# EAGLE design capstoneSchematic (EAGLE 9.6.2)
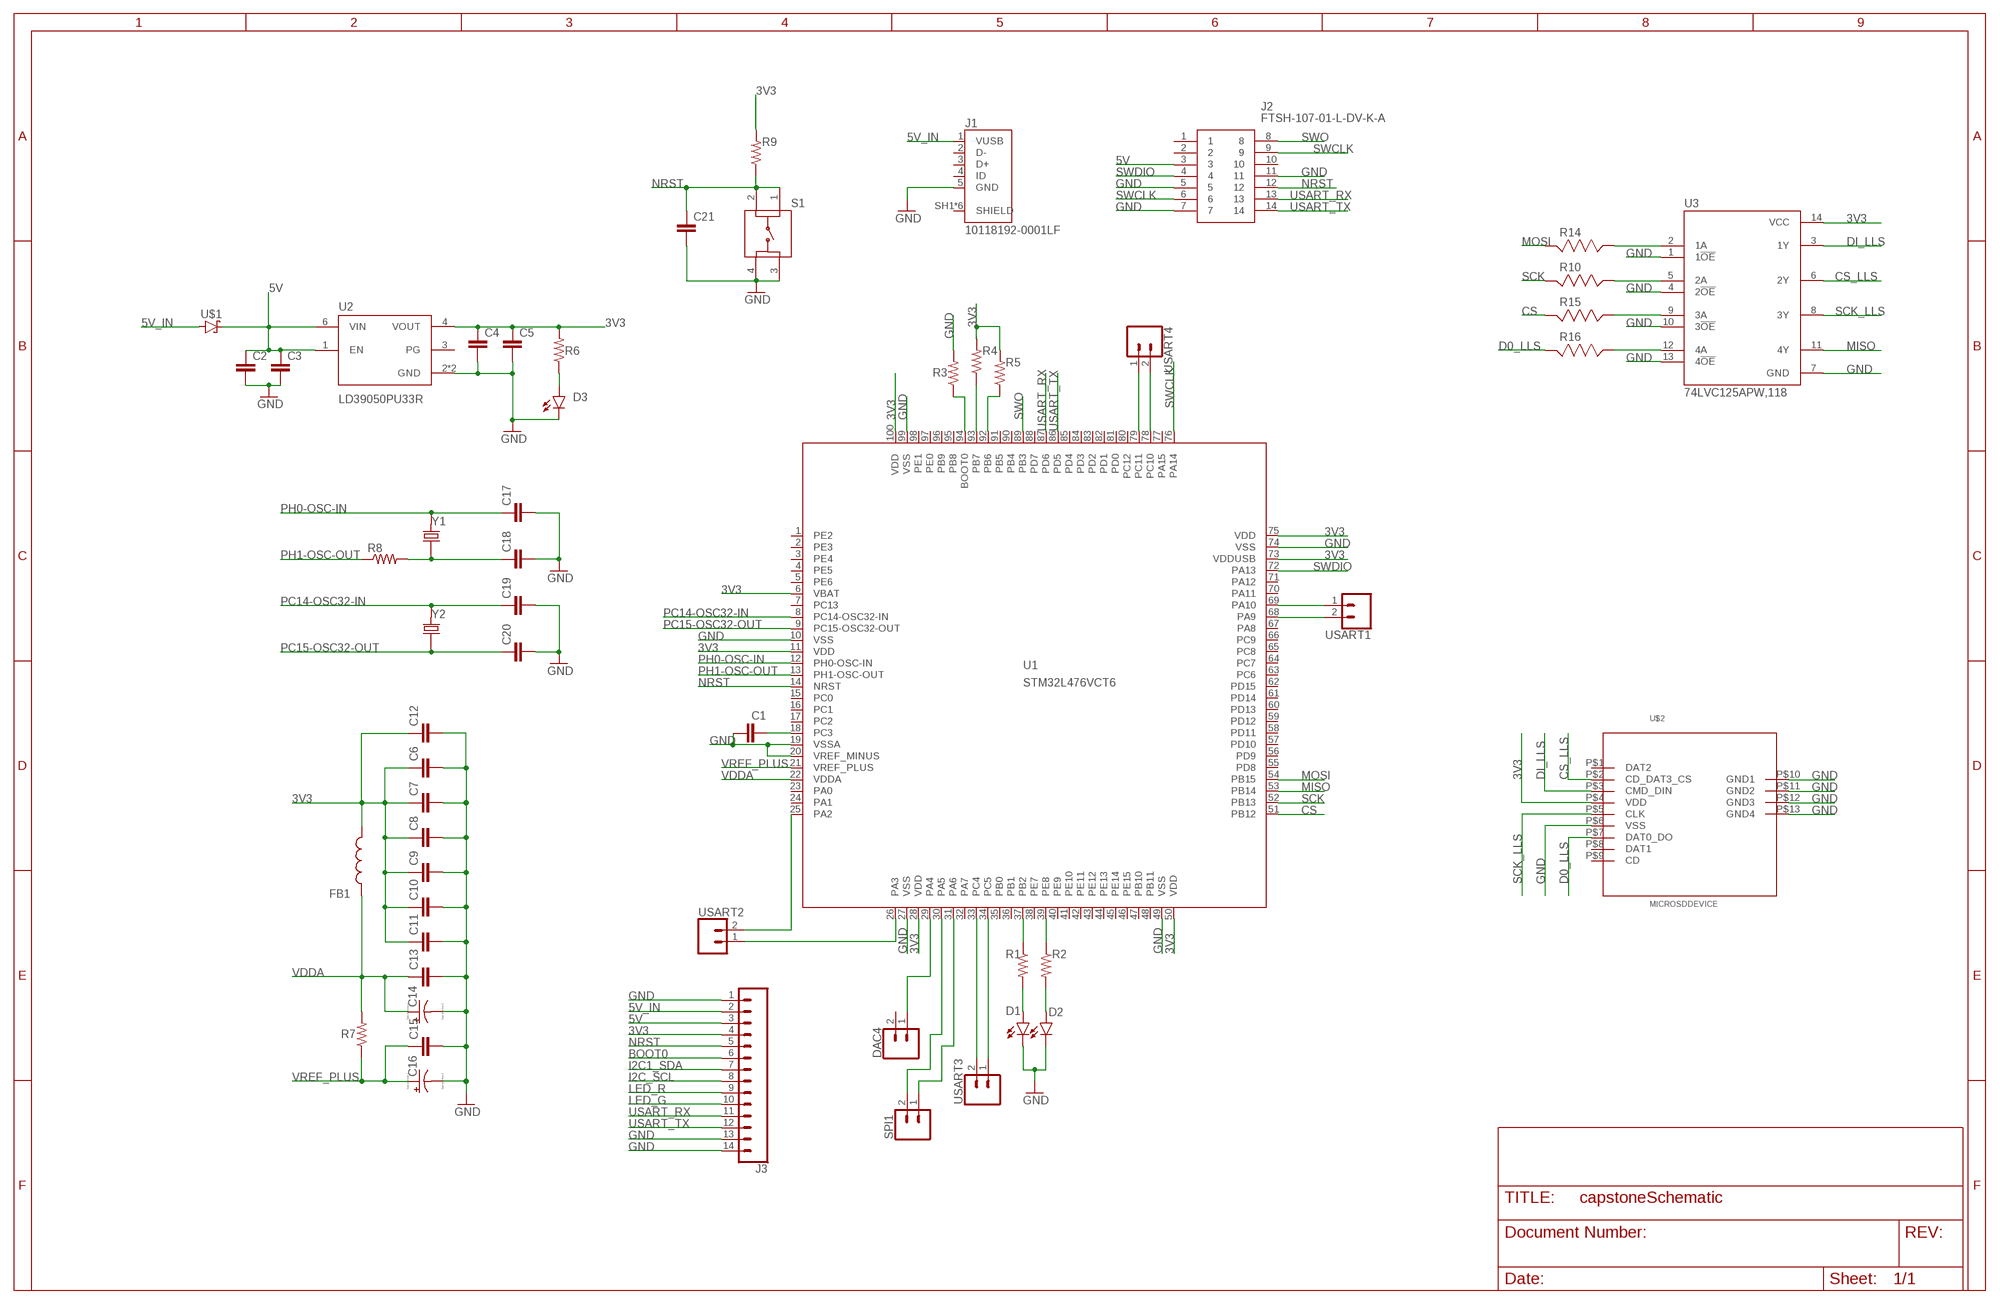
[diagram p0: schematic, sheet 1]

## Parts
C1  CC0603KRX5R7BB105  [CAPC1608X90]
C2  CC0603KRX5R7BB105  [CAPC1608X90]
C3  CC0402KRX7R7BB104  [CAPC1005X55N]
C4  CC0603KRX5R7BB105  [CAPC1608X90]
C5  CC0402KRX7R7BB104  [CAPC1005X55N]
C6  CC0402KRX7R7BB104  [CAPC1005X55N]
C7  CC0402KRX7R7BB104  [CAPC1005X55N]
C8  CC0402KRX7R7BB104  [CAPC1005X55N]
C9  CC0402KRX7R7BB104  [CAPC1005X55N]
C10  CC0402KRX7R7BB104  [CAPC1005X55N]
C11  CC0402KRX7R7BB104  [CAPC1005X55N]
C12  CC0603KRX5R7BB105  [CAPC1608X90]
C13  CC0402KRX7R7BB104  [CAPC1005X55N]
C14  TAJA105K016RNJ  [CAPPM3216X180N]
C15  CC0402KRX7R7BB104  [CAPC1005X55N]
C16  TAJA105K016RNJ  [CAPPM3216X180N]
C17  CC0402JRNPO9BN200  [CAPC1005X55N]
C18  CC0402JRNPO9BN200  [CAPC1005X55N]
C19  CC0402CRNPO9BN4R7  [CAPC1005X55N]
C20  CC0402CRNPO9BN4R7  [CAPC1005X55N]
C21  CC0402KRX7R7BB104  [CAPC1005X55N]
D1  SML-P12MTT86  [LED_SML-P11UTT86R]
D2  SML-P12MTT86  [LED_SML-P11UTT86R]
D3  SML-P12MTT86  [LED_SML-P11UTT86R]
DAC4  CONN_02  [1X02]
FB1  BK1608HS601-T  [BEADC1608X95N]
J1  10118192-0001LF  [AMPHENOL_10118192-0001LF]
J2  FTSH-107-01-L-DV-K-A  [FTSH10701LDVKA]
J3  CONN_14  [1X14]
R1  RC0402FR-071KL  [RESC1005X40N]
R2  RC0402FR-071KL  [RESC1005X40N]
R3  RC0402FR-071KL  [RESC1005X40N]
R4  RC0402FR-071KL  [RESC1005X40N]
R5  RC0402FR-071KL  [RESC1005X40N]
R6  RC0402FR-071KL  [RESC1005X40N]
R7  RC0402FR-071KL  [RESC1005X40N]
R8  RC0402FR-072KL  [RESC1005X40N]
R9  RC0402FR-0710KL  [RESC1005X40N]
R10  RC0402FR-073K3L  [RESC1005X40]
R14  RC0402FR-073K3L  [RESC1005X40]
R15  RC0402FR-073K3L  [RESC1005X40]
R16  RC0402FR-073K3L  [RESC1005X40]
S1  LL3301FF065QJ  [LL3301FF065QJ]
SPI1  CONN_02  [1X02]
U1  STM32L476VCT6  [LQFP100_14X14]
U2  LD39050PU33R  [SON95P300X300X100-7N]
U3  74LVC125APW,118  [IC_74LVC125APW,118]
U$1  STPS1L30A  [DIOM5226X223N]
U$2  MICROSDDEVICE  [MICROSD]
USART1  CONN_02  [1X02]
USART2  CONN_02  [1X02]
USART3  CONN_02  [1X02]
USART4  CONN_02  [1X02]
Y1  ABLS-8.000MHZ-B2-T  [XTAL_ABLS-8.000MHZ-B2-T]
Y2  ECS-.327-12.5-12QS-TR  [XTAL_ECS-.327-12.5-12QS-TR]

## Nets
3V3: C4.1 C5.1 C6.1 C7.1 C8.1 C9.1 C10.1 C11.1 C12.1 FB1.2 J3.4 R4.2 R5.2 R6.2 R9.2 U1.6(VBAT) U1.11(VDD) U1.28(VDD) U1.50(VDD) U1.73(VDDUSB) U1.75(VDD) U1.100(VDD) U2.4(VOUT) U3.14(VCC) U$2.P$4(VDD)
5V: C2.1 C3.1 J2.3 J3.3 U2.1(EN) U2.6(VIN) U$1.1(C)
5V_IN: J1.1(VUSB) J3.2 U$1.2(A)
BOOT0: J3.6
CS: R15.1 U1.51(PB12)
CS_LLS: U3.6(2Y) U$2.P$2(CD_DAT3_CS)
D0_LLS: R16.1 U$2.P$7(DAT0_DO)
DI_LLS: U3.3(1Y) U$2.P$3(CMD_DIN)
GND: C1.1 C2.2 C3.2 C4.2 C5.2 C6.2 C7.2 C8.2 C9.2 C10.2 C11.2 C12.2 C13.2 C14.C(-) C15.2 C16.C(-) C17.2 C18.2 C19.2 C20.2 C21.2 D1.C D2.C D3.C J1.5(GND) J2.5 J2.7 J2.11 J3.1 J3.13 J3.14 R3.2 S1.3 S1.4 U1.10(VSS) U1.19(VSSA) U1.20(VREF_MINUS) U1.27(VSS) U1.49(VSS) U1.74(VSS) U1.99(VSS) U2.2(GND) U2.7(GND) U3.1(1!OE) U3.4(2!OE) U3.7(GND) U3.10(3!OE) U3.13(4!OE) U$2.P$6(VSS) U$2.P$10(GND1) U$2.P$11(GND2) U$2.P$12(GND3) U$2.P$13(GND4)
I2C1_SDA: J3.7
I2C_SCL: J3.8
LED_G: J3.10
LED_R: J3.9
MISO: U1.53(PB14) U3.11(4Y)
MOSI: R14.1 U1.54(PB15)
N$1: R2.1 U1.39(PE8)
N$2: R1.1 U1.37(PB2)
N$3: D1.A R1.2
N$4: D2.A R2.2
N$5: R3.1 U1.94(BOOT0)
N$6: R4.1 U1.93(PB7)
N$7: R5.1 U1.92(PB6)
N$8: D3.A R6.1
N$9: U1.33(PC4) USART3.2
N$10: C1.2 U1.18(PC3)
N$11: U1.34(PC5) USART3.1
N$12: C18.1 R8.2 Y1.1
N$13: R14.2 U3.2(1A)
N$14: U1.78(PC10) USART4.2
N$15: DAC4.1 U1.29(PA4)
N$16: U1.79(PC11) USART4.1
N$17: SPI1.2 U1.30(PA5)
N$18: SPI1.1 U1.31(PA6)
N$19: U1.69(PA10) USART1.1
N$20: U1.68(PA9) USART1.2
N$22: U1.25(PA2) USART2.2
N$23: U1.26(PA3) USART2.1
N$24: R10.2 U3.5(2A)
N$25: R15.2 U3.9(3A)
N$26: R16.2 U3.12(4A)
NRST: C21.1 J2.12 J3.5 R9.1 S1.1 S1.2 U1.14(NRST)
PC14-OSC32-IN: C19.1 U1.8(PC14-OSC32-IN) Y2.2
PC15-OSC32-OUT: C20.1 U1.9(PC15-OSC32-OUT) Y2.1
PH0-OSC-IN: C17.1 U1.12(PH0-OSC-IN) Y1.2
PH1-OSC-OUT: R8.1 U1.13(PH1-OSC-OUT)
SCK: R10.1 U1.52(PB13)
SCK_LLS: U3.8(3Y) U$2.P$5(CLK)
SWCLK: J2.6 J2.9 U1.76(PA14)
SWDIO: J2.4 U1.72(PA13)
SWO: J2.8 U1.89(PB3)
USART_RX: J2.13 J3.11 U1.87(PD6)
USART_TX: J2.14 J3.12 U1.86(PD5)
VDDA: C13.1 C14.A(+) FB1.1 R7.2 U1.22(VDDA)
VREF_PLUS: C15.1 C16.A(+) R7.1 U1.21(VREF_PLUS)
Unconnected: DAC4.2 J1.2(D-) J1.3(D+) J1.4(ID) J1.SH1(SHIELD) J1.SH2(SHIELD) J1.SH3(SHIELD) J1.SH4(SHIELD) J1.SH5(SHIELD) J1.SH6(SHIELD) J2.1 J2.2 J2.10 U1.1(PE2) U1.2(PE3) U1.3(PE4) U1.4(PE5) U1.5(PE6) U1.7(PC13) U1.15(PC0) U1.16(PC1) U1.17(PC2) U1.23(PA0) U1.24(PA1) U1.32(PA7) U1.35(PB0) U1.36(PB1) U1.38(PE7) U1.40(PE9) U1.41(PE10) U1.42(PE11) U1.43(PE12) U1.44(PE13) U1.45(PE14) U1.46(PE15) U1.47(PB10) U1.48(PB11) U1.55(PD8) U1.56(PD9) U1.57(PD10) U1.58(PD11) U1.59(PD12) U1.60(PD13) U1.61(PD14) U1.62(PD15) U1.63(PC6) U1.64(PC7) U1.65(PC8) U1.66(PC9) U1.67(PA8) U1.70(PA11) U1.71(PA12) U1.77(PA15) U1.80(PC12) U1.81(PD0) U1.82(PD1) U1.83(PD2) U1.84(PD3) U1.85(PD4) U1.88(PD7) U1.90(PB4) U1.91(PB5) U1.95(PB8) U1.96(PB9) U1.97(PE0) U1.98(PE1) U2.3(PG) U$2.P$1(DAT2) U$2.P$8(DAT1) U$2.P$9(CD)

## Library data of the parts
C1 C2 C4 C12 = ce-capstone:CC0603KRX5R7BB105: CAPACITOR CERAMIC, 1µF, 10V, X5R, 0603; Dielectric Characteristic:X5R; Capacitance:1µF; Capacitance Tolerance:± 10%; Voltage Rating:16V; Temperature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; DESCRIPTION: 1µF ±10% 16V Ceramic Capacitor X5R 0603 _1608 Metric_; DIGI-KEY_PART_NUMBER: 311-1444-1-ND; DIGI-KEY_PURCHASE_URL: https://www.digikey.com/product-detail/en/yageo/CC0603KRX5R7BB105/311-1444-1-ND/2833750?utm_source=snapeda&utm_medium=aggregator&utm_campaign=symbol; MF: Yageo; MP: CC0603KRX5R7BB105; PACKAGE: 0603 Yageo
C3 C5-C11 C13 C15 C21 = ce-capstone:CC0402KRX7R7BB104: .1UF 16V 10% 0402; DESCRIPTION: 0.1µF ±10% 16V Ceramic Capacitor X7R 0402 _1005 Metric_; DIGI-KEY_PART_NUMBER: 311-1338-1-ND; DIGI-KEY_PURCHASE_URL: https://www.digikey.com/product-detail/en/yageo/CC0402KRX7R7BB104/311-1338-1-ND/2103122?utm_source=snapeda&utm_medium=aggregator&utm_campaign=symbol; MF: Yageo; MP: CC0402KRX7R7BB104; PACKAGE: 0402 Yageo
C14 C16 = ce-capstone:TAJA105K016RNJ: Capacitor tantalum TAJ 1206 1uF 16V AVX 1uF SMD Solid MnO2 Tantalum Electrolytic Capacitor, 16 V dc +/-10%, TAJ Series; ALLIED_NUMBER: 70474975; ALLIED_PRICE-STOCK: https://www.alliedelec.com/avx-taja105k016r/70474975/; DESCRIPTION: Capacitor tantalum TAJ 1206 1uF 16V AVX 1uF SMD Solid MnO2 Tantalum Electrolytic Capacitor, 16 V dc +/-10%, TAJ Series; HEIGHT: 1.8mm; MANUFACTURER_NAME: AVX; MANUFACTURER_PART_NUMBER: TAJA105K016RNJ; MOUSER_PART_NUMBER: 581-TAJA105K016RNJ; MOUSER_PRICE-STOCK: https://www.mouser.com/Search/Refine.aspx?Keyword=581-TAJA105K016R; RS_PART_NUMBER: 6992804P; RS_PRICE-STOCK: http://uk.rs-online.com/web/p/products/6992804P
C17 C18 = ce-capstone:CC0402JRNPO9BN200: CAPACITOR CERAMIC 20PF 50V, C0G, 0402; Dielectric Characteristic:C0G / NP0; Capacitance:20pF; Capacitance Tolerance:± 5%; Voltage Rating:50V; Capacitor Case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; DESCRIPTION: 20pF ±5% 50V Ceramic Capacitor C0G, NP0 0402 _1005 Metric_; DIGI-KEY_PART_NUMBER: 311-1417-1-ND; DIGI-KEY_PURCHASE_URL: https://www.digikey.com/product-detail/en/yageo/CC0402JRNPO9BN200/311-1417-1-ND/2833723?utm_source=snapeda&utm_medium=aggregator&utm_campaign=symbol; MF: Yageo; MP: CC0402JRNPO9BN200; PACKAGE: 0402 Yageo
C19 C20 = ce-capstone:CC0402CRNPO9BN4R7: 0402 4.7 pF 50 V ±0.25 pF Tolerance NP0 SMT Multilayer Ceramic Capacitor; DESCRIPTION: 4.7pF ±0.25pF 50V Ceramic Capacitor C0G, NP0 0402 _1005 Metric_; DIGI-KEY_PART_NUMBER: 311-1367-1-ND; DIGI-KEY_PURCHASE_URL: https://www.digikey.com/product-detail/en/yageo/CC0402CRNPO9BN4R7/311-1367-1-ND/2103151?utm_source=snapeda&utm_medium=aggregator&utm_campaign=symbol; MF: Yageo; MP: CC0402CRNPO9BN4R7; PACKAGE: 0402 Yageo
D1-D3 = ce-capstone:SML-P12MTT86: SML-P1 Series Red 0402 Clear 60 mcd 2 V Surface Mount PICOLED LED; AVAILABILITY: Unavailable; DESCRIPTION: Green 572nm LED Indication - Discrete 2V 0402 _1006 Metric_; MF: Rohm; MP: SML-P12MTT86; PACKAGE: 0402 Rohm; PRICE: None
DAC4 SPI1 USART1-USART4 = SparkFun-Connectors:CONN_02: Multi connection point. Often used as Generic Header-pin footprint for 0.1 inch spaced/style header connections
FB1 = ce-capstone:BK1608HS601-T: Ferrite Chip Bead(Lead Free); DESCRIPTION: Ferrite Chip Bead(Lead Free); HEIGHT: 0.95mm; MANUFACTURER_NAME: Taiyo Yuden; MANUFACTURER_PART_NUMBER: BK1608HS601-T
J1 = ce-capstone:10118192-0001LF: Single Port 5 Contact Horizontal Right Angle Shielded Micro B USB 2.0 Connector; AVAILABILITY: Unavailable; DESCRIPTION: USB - micro B USB 2.0 Receptacle Connector 5 Position Surface Mount, Right Angle; MF: Amphenol ICC; MP: 10118192-0001LF; PACKAGE: None; PRICE: None
J2 = ce-capstone:FTSH-107-01-L-DV-K-A: Headers & Wire Housings .050" Micro Terminal Strip Source: Datasheet; DESCRIPTION: Headers & Wire Housings .050" Micro Terminal Strip; HEIGHT: 5.97mm; MANUFACTURER_NAME: SAMTEC; MANUFACTURER_PART_NUMBER: FTSH-107-01-L-DV-K-A; MOUSER_PART_NUMBER: 200-FTSH10701LDVKA; MOUSER_PRICE-STOCK: https://www.mouser.com/Search/Refine.aspx?Keyword=200-FTSH10701LDVKA
J3 = SparkFun-Connectors:CONN_14: Multi connection point. Often used as Generic Header-pin footprint for 0.1 inch spaced/style header connections On any of the 0.1 inch spaced packages, you can populate with these: Break Away Headers - Straight (PRT-00116) Break Away Male Headers - Right Angle (PRT-00553) Female Headers (PRT-00115)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
R1-R7 = ce-capstone:RC0402FR-071KL: RES SMD 1k OHM 1% 1/16W 0402; DESCRIPTION: 510 Ohms ±1% 0.063W, 1/16W Chip Resistor 0402 _1005 Metric_ Moisture Resistant Thick Film; DIGI-KEY_PART_NUMBER: 311-510LRCT-ND; DIGI-KEY_PURCHASE_URL: https://www.digikey.com/product-detail/en/yageo/RC0402FR-07510RL/311-510LRCT-ND/729579?utm_source=snapeda&utm_medium=aggregator&utm_campaign=symbol; MF: Yageo; MP: RC0402FR-07510RL; PACKAGE: 1005 Panasonic Electronic Components
R8 = ce-capstone:RC0402FR-072KL: RES SMD 2k OHM 1% 1/16W 0402; DESCRIPTION: 510 Ohms ±1% 0.063W, 1/16W Chip Resistor 0402 _1005 Metric_ Moisture Resistant Thick Film; DIGI-KEY_PART_NUMBER: 311-510LRCT-ND; DIGI-KEY_PURCHASE_URL: https://www.digikey.com/product-detail/en/yageo/RC0402FR-07510RL/311-510LRCT-ND/729579?utm_source=snapeda&utm_medium=aggregator&utm_campaign=symbol; MF: Yageo; MP: RC0402FR-07510RL; PACKAGE: 1005 Panasonic Electronic Components
R9 = ce-capstone:RC0402FR-0710KL: RES SMD 10k OHM 1% 1/16W 0402; DESCRIPTION: 510 Ohms ±1% 0.063W, 1/16W Chip Resistor 0402 _1005 Metric_ Moisture Resistant Thick Film; DIGI-KEY_PART_NUMBER: 311-510LRCT-ND; DIGI-KEY_PURCHASE_URL: https://www.digikey.com/product-detail/en/yageo/RC0402FR-07510RL/311-510LRCT-ND/729579?utm_source=snapeda&utm_medium=aggregator&utm_campaign=symbol; MF: Yageo; MP: RC0402FR-07510RL; PACKAGE: 1005 Panasonic Electronic Components
R10 R14-R16 = RC0402FR-073K3L:RC0402FR-073K3L: RC Series 0402 0.063 W 3.3 kOhms ±1% ±100 ppm/°C SMT Thick Film Chip Resistor; MANUFACTURER: YAGEO
S1 = ce-capstone:LL3301FF065QJ: Pushbutton Switches 50mA 12VDC F065 7.0mm J-Lead Source: Datasheet; DESCRIPTION: Pushbutton Switches 50mA 12VDC F065 7.0mm J-Lead; HEIGHT: 7.3mm; MANUFACTURER_NAME: E-Switch; MANUFACTURER_PART_NUMBER: LL3301FF065QJ; MOUSER_PART_NUMBER: 612-LL3301FF065QJ; MOUSER_PRICE-STOCK: https://www.mouser.com/Search/Refine.aspx?Keyword=612-LL3301FF065QJ
U1 = ce-capstone:STM32L476V*: STM32L476VX LQFP100 Datasheet STM32L476XX; FARNELL: 2518171; FLASH: 256kB; SRAM: 128kB
U2 = ce-capstone:LD39050PU33R: LD39050 Series 500 mA 3.3 V Fixed Low Noise LDO Voltage Regulator - DFN-6; AVAILABILITY: Unavailable; DESCRIPTION: Linear Voltage Regulator IC 1 Output 500mA 6-DFN _3x3_; MF: STMicroelectronics; MP: LD39050PU33R; PACKAGE: DFN-6 STMicroelectronics; PRICE: None
U3 = 74LVC125APW_118:74LVC125APW,118: Check availability Check availability Check availability; AVAILABILITY: In Stock; CHECK_PRICES: https://www.snapeda.com/parts/74LVC125APW,118/Nexperia/view-part/?ref=eda; DESCRIPTION: Buffer, Non-Inverting 4 Element 1 Bit per Element 3-State Output 14-TSSOP; MF: Nexperia USA Inc.; MP: 74LVC125APW,118; PACKAGE: TSSOP14-14 Nexperia USA Inc.; PRICE: None; PURCHASE-URL: https://www.snapeda.com/api/url_track_click_mouser/?unipart_id=5248541&manufacturer=Nexperia USA Inc.&part_name=74LVC125APW,118&search_term=None; SNAPEDA_LINK: https://www.snapeda.com/parts/74LVC125APW,118/Nexperia/view-part/?ref=snap
U$1 = ce-capstone:STPS1L30A
U$2 = MicroSDFootprint:MICROSDDEVICE
Y1 = ce-capstone:ABLS-8.000MHZ-B2-T: Crystal 8MHz Â±20ppm (Tol) Â±50ppm (Stability) 18pF FUND 80Ohm 2-Pin HC-49/US SMD T/R; AVAILABILITY: Unavailable; DESCRIPTION: 8MHz ±20ppm Crystal 18pF 80 Ohms HC-49/US; MF: Abracon LLC; MP: ABLS-8.000MHZ-B2; PACKAGE: HC-49/US Abracon LLC; PRICE: None
Y2 = ce-capstone:ECS-.327-12.5-12QS-TR: SMD CRYSTAL 32.768 KHz; AVAILABILITY: Unavailable; DESCRIPTION: 32.768kHz ±20ppm Crystal 12.5pF 90 kOhms 2-SMD, No Lead; MF: ECS Inc.; MP: ECS-.327-12.5-12QS-TR; PACKAGE: SMD-2 ECS International; PRICE: None

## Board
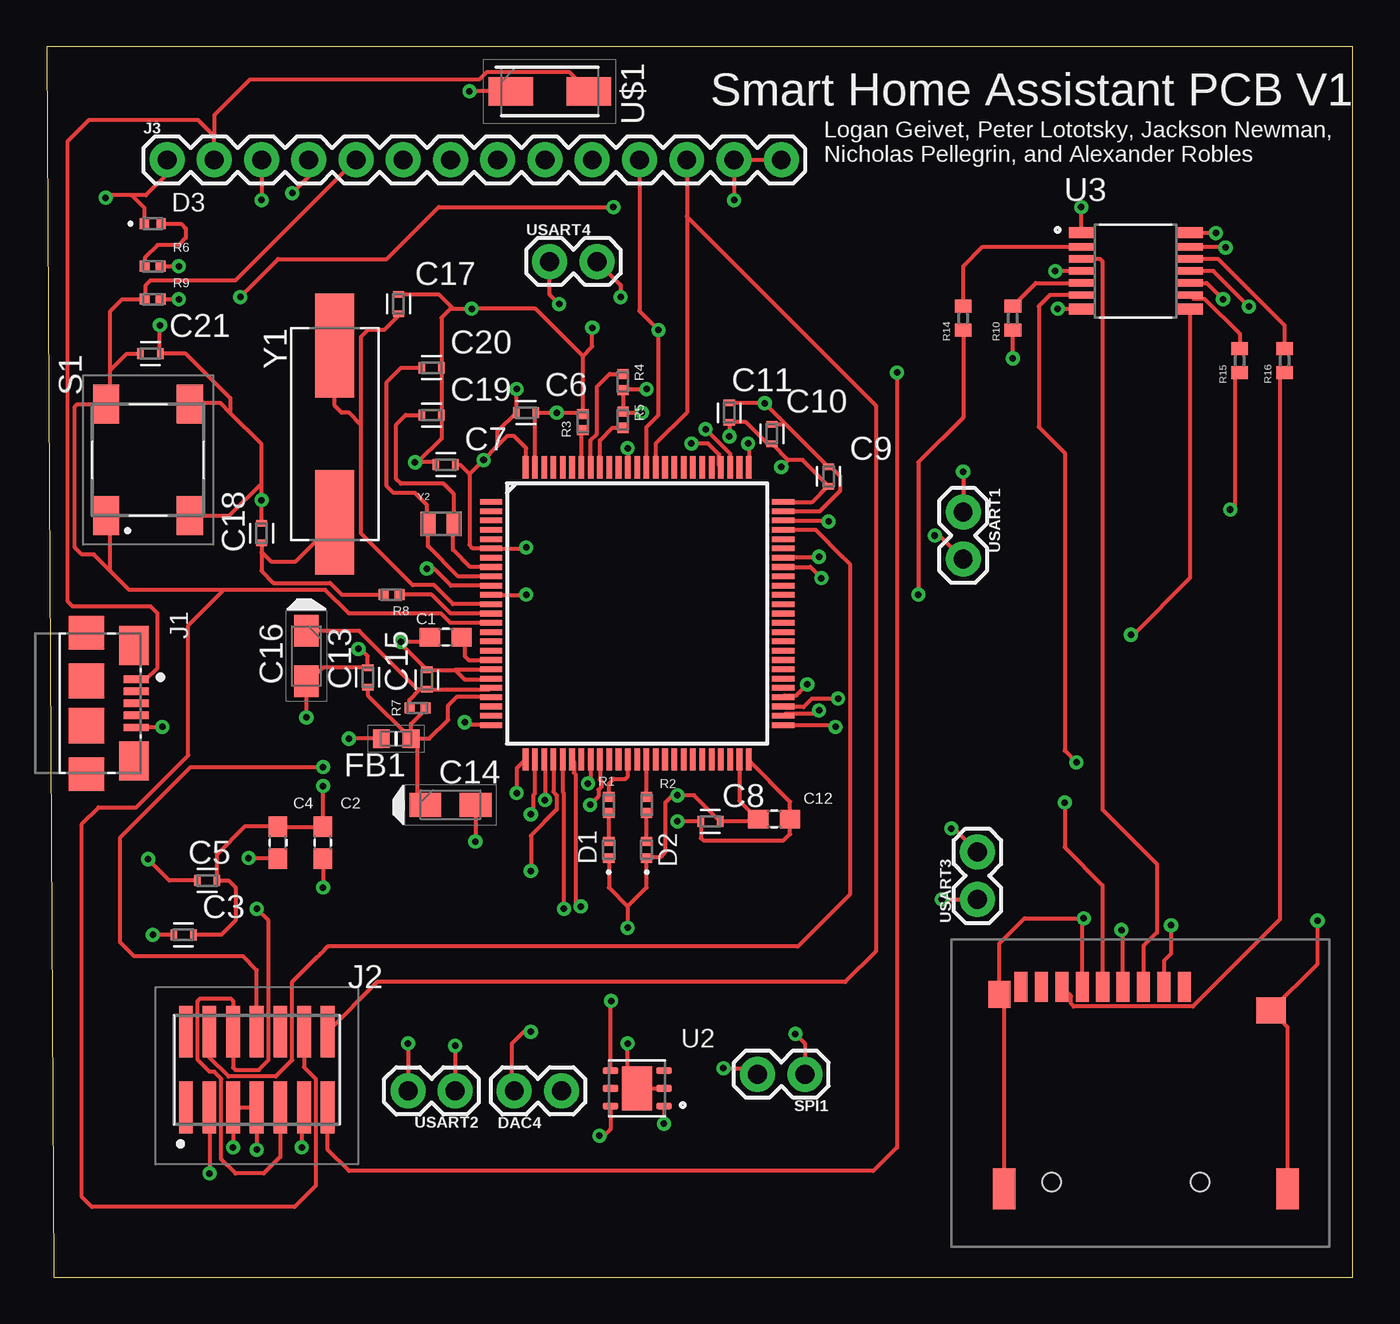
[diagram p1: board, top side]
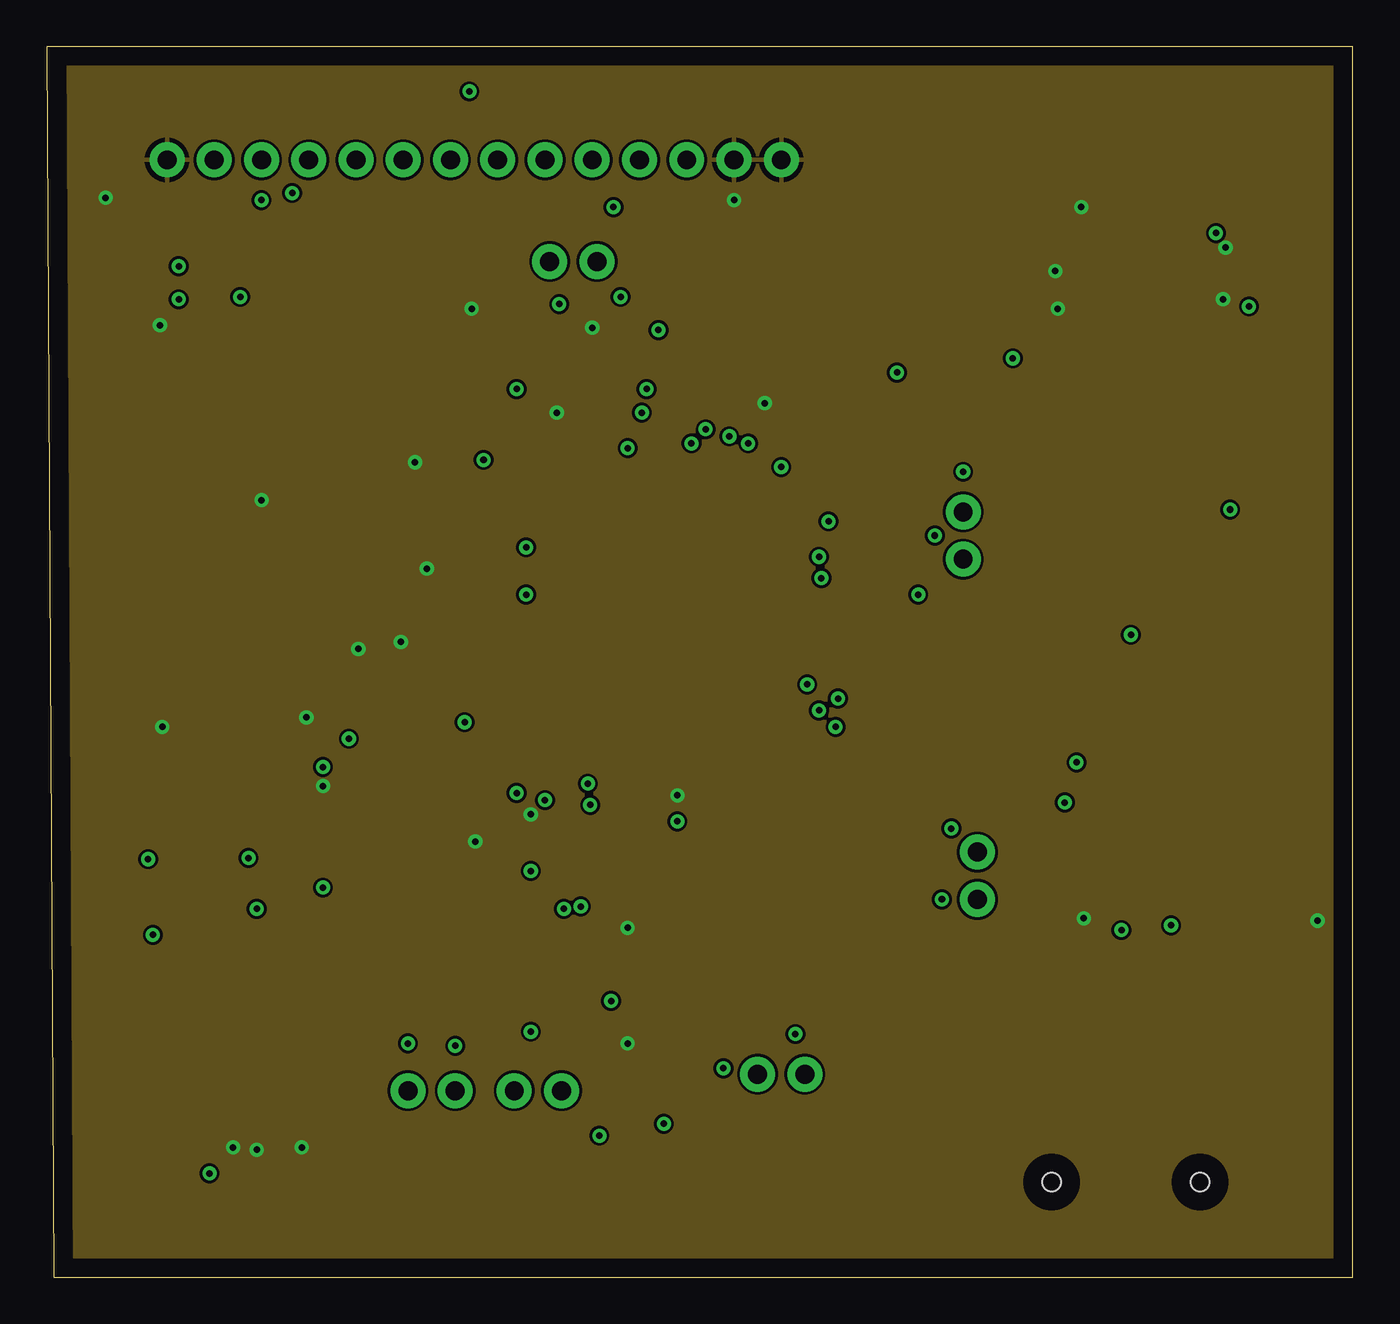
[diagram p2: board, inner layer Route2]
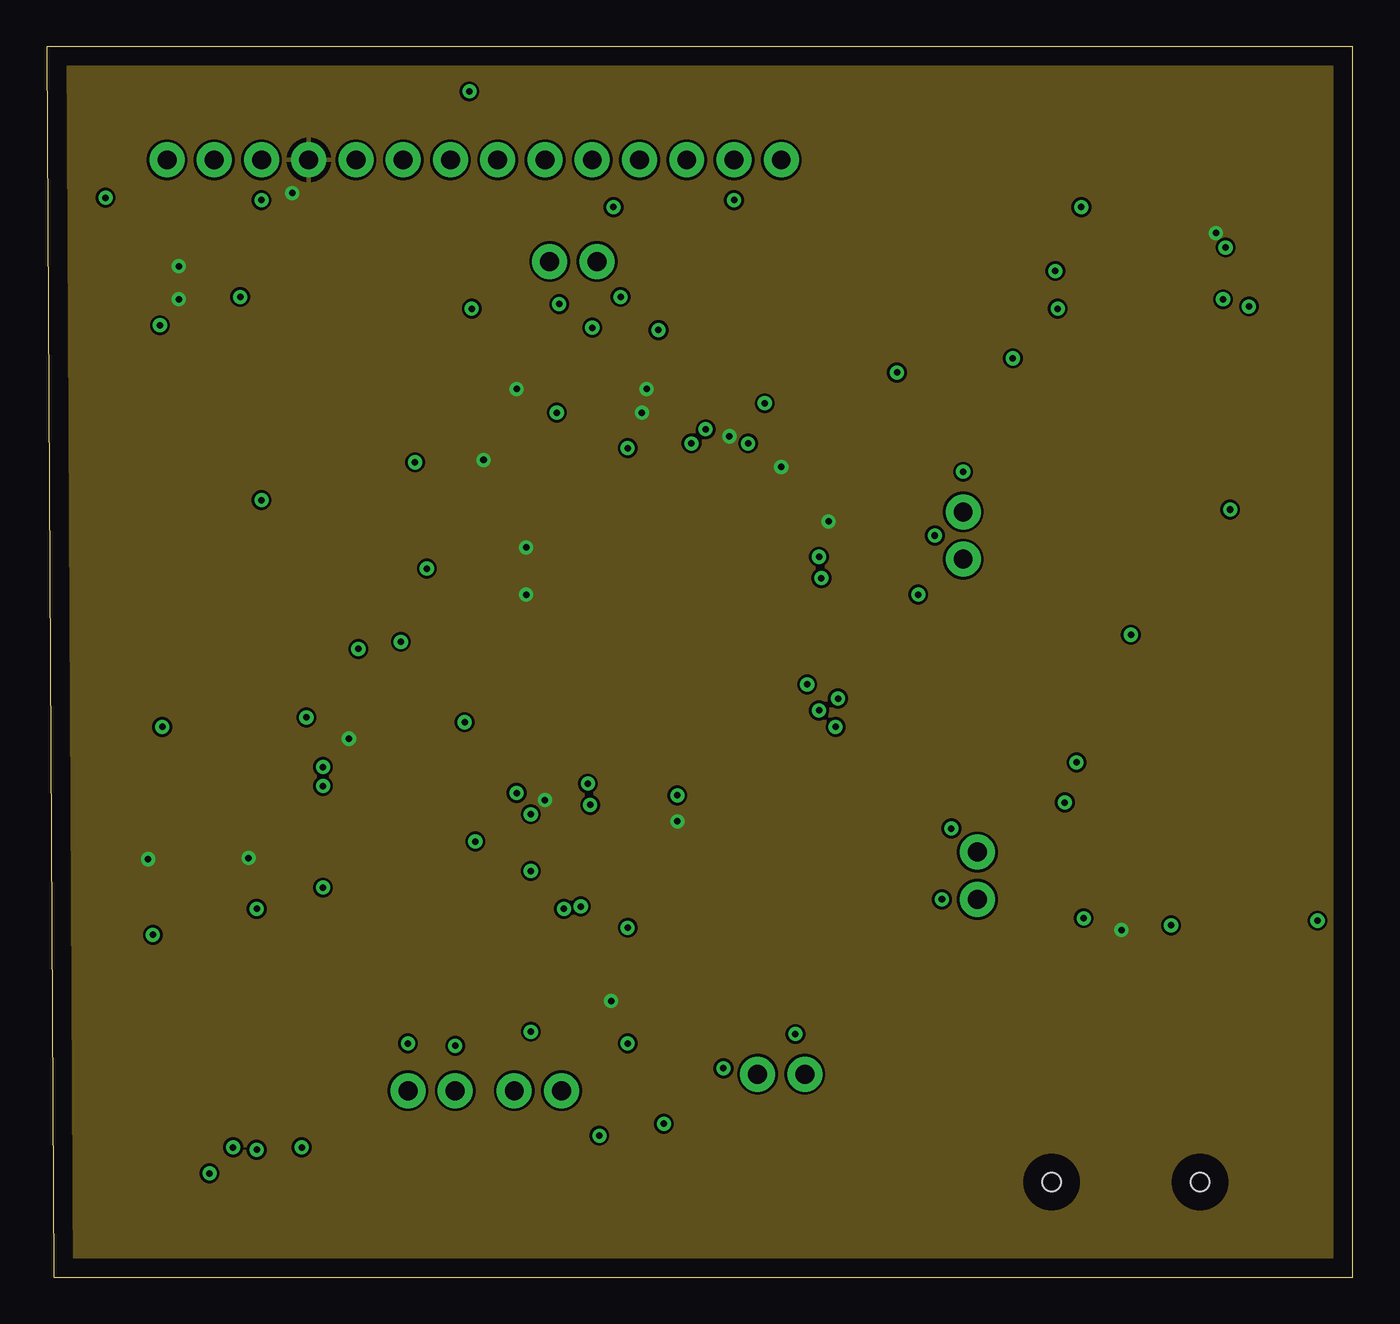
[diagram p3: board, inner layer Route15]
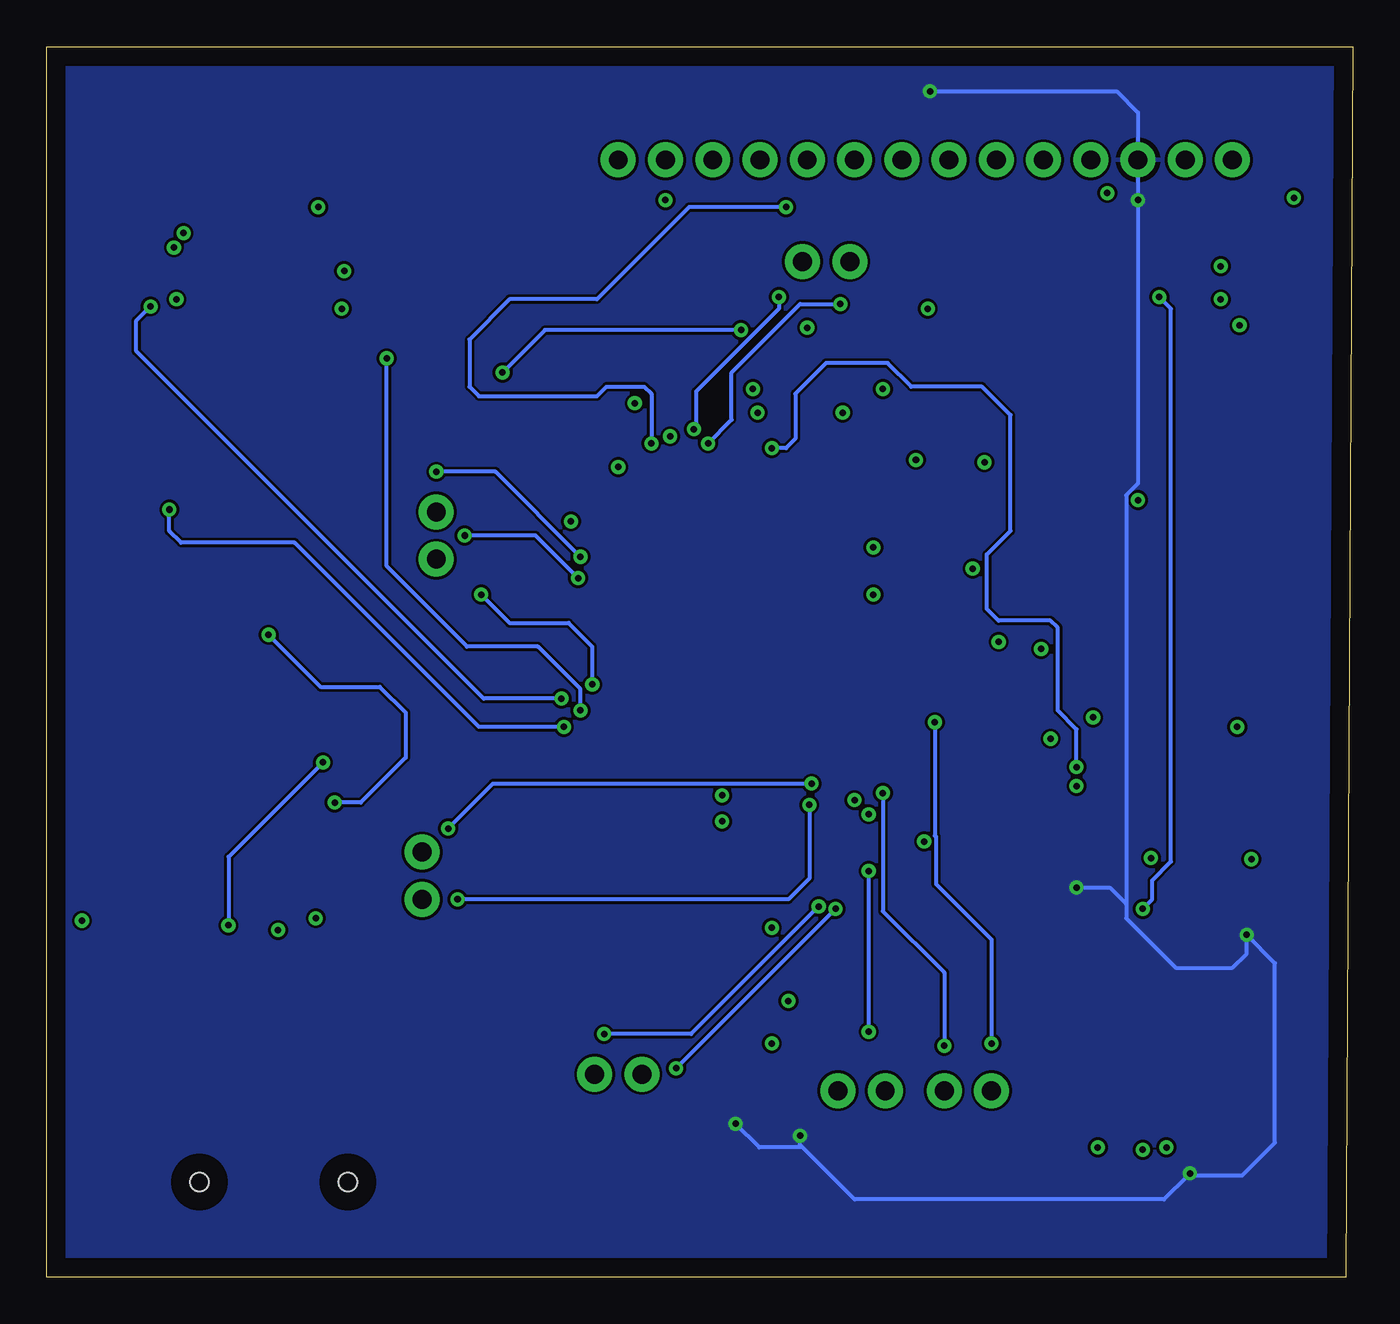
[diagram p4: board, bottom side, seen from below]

Size 70.23 x 66.17 mm. Coordinates in mm from the lower left corner, seen from the top.
Outline: 0.38,0 70.23,0 70.23,66.17 0,66.17 0.38,0
Copper layers (1+2*15+16): Top 0.035mm / dielectric 1.5mm / Route2 0.035mm / dielectric 0.15mm / Route15 0.035mm / dielectric 0.2mm / Bottom 0.035mm
Design rules "default *": minimum track width 8mil, minimum drill 0.35mm, track to track 6mil, track to pad 6mil, pad to pad 6mil, via to via 6mil, smd to smd 6mil, copper to edge 40mil, drill to drill 6mil, minimum pad ring 10mil, minimum via ring 8mil, stop-mask expansion 4mil, vias tented up to drill 0mil, thermal gap 10mil

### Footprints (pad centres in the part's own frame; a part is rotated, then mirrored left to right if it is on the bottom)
CAPC1608X90 = smd 1.1 x 1: 1 -0.85,0; 2 0.85,0
CAPC1005X55N = smd 0.35 x 0.6: 1 -0.525,0; 2 0.525,0
CAPPM3216X180N = smd 1.7 x 1.3: A -1.35,0; C 1.35,0
LED_SML-P11UTT86R = smd 0.5 x 0.6: A 0.45,0; C -0.45,0
1X02 = drill 1.016 pad 1.88: 1 0,0; 2 2.54,0
BEADC1608X95N = smd 0.9 x 1: 1 -0.8,0; 2 0.8,0
AMPHENOL_10118192-0001LF = smd 0.4 x 1.35: 1 -1.3,0; 2 -0.65,0; 3 0,0; 4 0.65,0; 5 1.3,0 | smd 2.1 x 1.6: SH1 -3.1,-0.125; SH2 3.1,-0.125 | smd 1.8 x 1.9: SH3 -3.8,-2.675; SH6 3.8,-2.675 | smd 1.9 x 1.9: SH4 -1.2,-2.675; SH5 1.2,-2.675
FTSH10701LDVKA = smd 0.74 x 2.79: 1 -3.81,-2.035; 2 -3.81,2.035; 3 -2.54,-2.035; 4 -2.54,2.035; 5 -1.27,-2.035; 6 -1.27,2.035; 7 0,-2.035; 8 0,2.035; 9 1.27,-2.035; 10 1.27,2.035; 11 2.54,-2.035; 12 2.54,2.035; 13 3.81,-2.035; 14 3.81,2.035
1X14 = drill 1.016 pad 1.88: 1 0,0; 2 2.54,0; 3 5.08,0; 4 7.62,0; 5 10.16,0; 6 12.7,0; 7 15.24,0; 8 17.78,0; 9 20.32,0; 10 22.86,0; 11 25.4,0; 12 27.94,0; 13 30.48,0; 14 33.02,0
RESC1005X40N = smd 0.54 x 0.6: 1 -0.432,0; 2 0.432,0
RESC1005X40 = smd 0.7 x 0.9: 1 -0.65,0; 2 0.65,0
LL3301FF065QJ = smd 2.1 x 1.4: 1 -3,2.25; 2 3,2.25; 3 -3,-2.25; 4 3,-2.25
LQFP100_14X14 = smd 1.2 x 0.3: 1 -7.85,6; 2 -7.85,5.5; 3 -7.85,5; 4 -7.85,4.5; 5 -7.85,4; 6 -7.85,3.5; 7 -7.85,3; 8 -7.85,2.5; 9 -7.85,2; 10 -7.85,1.5; 11 -7.85,1; 12 -7.85,0.5; 13 -7.85,0; 14 -7.85,-0.5; 15 -7.85,-1; 16 -7.85,-1.5; 17 -7.85,-2; 18 -7.85,-2.5; 19 -7.85,-3; 20 -7.85,-3.5; 21 -7.85,-4; 22 -7.85,-4.5; 23 -7.85,-5; 24 -7.85,-5.5; 25 -7.85,-6; 51 7.85,-6; 52 7.85,-5.5; 53 7.85,-5; 54 7.85,-4.5; 55 7.85,-4; 56 7.85,-3.5; 57 7.85,-3; 58 7.85,-2.5; 59 7.85,-2; 60 7.85,-1.5; 61 7.85,-1; 62 7.85,-0.5; 63 7.85,0; 64 7.85,0.5; 65 7.85,1; 66 7.85,1.5; 67 7.85,2; 68 7.85,2.5; 69 7.85,3; 70 7.85,3.5; 71 7.85,4; 72 7.85,4.5; 73 7.85,5; 74 7.85,5.5; 75 7.85,6 | smd 0.3 x 1.2: 26 -6,-7.85; 27 -5.5,-7.85; 28 -5,-7.85; 29 -4.5,-7.85; 30 -4,-7.85; 31 -3.5,-7.85; 32 -3,-7.85; 33 -2.5,-7.85; 34 -2,-7.85; 35 -1.5,-7.85; 36 -1,-7.85; 37 -0.5,-7.85; 38 0,-7.85; 39 0.5,-7.85; 40 1,-7.85; 41 1.5,-7.85; 42 2,-7.85; 43 2.5,-7.85; 44 3,-7.85; 45 3.5,-7.85; 46 4,-7.85; 47 4.5,-7.85; 48 5,-7.85; 49 5.5,-7.85; 50 6,-7.85; 76 6,7.85; 77 5.5,7.85; 78 5,7.85; 79 4.5,7.85; 80 4,7.85; 81 3.5,7.85; 82 3,7.85; 83 2.5,7.85; 84 2,7.85; 85 1.5,7.85; 86 1,7.85; 87 0.5,7.85; 88 0,7.85; 89 -0.5,7.85; 90 -1,7.85; 91 -1.5,7.85; 92 -2,7.85; 93 -2.5,7.85; 94 -3,7.85; 95 -3.5,7.85; 96 -4,7.85; 97 -4.5,7.85; 98 -5,7.85; 99 -5.5,7.85; 100 -6,7.85
SON95P300X300X100-7N = smd 0.84 x 0.4: 1 -1.435,0.95; 2 -1.435,0; 3 -1.435,-0.95; 4 1.435,-0.95; 5 1.435,0; 6 1.435,0.95 | smd 1.625 x 2.365: 7 0,0
IC_74LVC125APW,118 = smd 1.35 x 0.6: 1 -2.925,2.05; 7 -2.925,-2.05; 8 2.925,-2.05; 14 2.925,2.05 | smd 1.35 x 0.4: 2 -2.925,1.3; 3 -2.925,0.65; 4 -2.925,0; 5 -2.925,-0.65; 6 -2.925,-1.3; 9 2.925,-1.3; 10 2.925,-0.65; 11 2.925,0; 12 2.925,0.65; 13 2.925,1.3
DIOM5226X223N = smd 2.4 x 1.55: 1 -2.1,0; 2 2.1,0
MICROSD = smd 1.6 x 0.7: P$1 -3.81,1.1; P$2 -3.81,0; P$3 -3.81,-1.1; P$4 -3.81,-2.2; P$5 -3.81,-3.3; P$6 -3.81,-4.4; P$7 -3.81,-5.5; P$8 -3.81,-6.6; P$9 -3.81,-7.7 | smd 1.45 x 1.2: P$10 -3.41,-8.85 | smd 1.4 x 1.6: P$11 -2.54,5.75 | smd 2.2 x 1.2: P$12 7.06,6.65; P$13 7.06,-8.59 | hole 1: 6.69,1.95; 6.69,-6.03
XTAL_ABLS-8.000MHZ-B2-T = smd 5.6 x 2.1: 1 -4.75,0; 2 4.75,0
XTAL_ECS-.327-12.5-12QS-TR = smd 0.8 x 1.3: 1 -0.7,0; 2 0.7,0

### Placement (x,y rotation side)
C1  21.46,34.42 0 top
C2  14.86,23.37 90 top
C3  7.37,18.41 0 top
C4  12.45,23.37 90 top
C5  8.64,21.34 0 top
C6  25.78,46.48 0 top
C7  21.46,43.69 180 top
C8  35.69,24.51 0 top
C9  42.04,43.05 90 top
C10  38.99,45.34 90 top
C11  36.7,46.48 90 top
C12  39.12,24.64 180 top
C13  17.27,32.26 90 top
C14  21.72,25.4 0 top
C15  20.45,32.13 90 top
C16  13.97,33.4 270 top
C17  18.92,52.32 90 top
C18  11.56,40.01 90 top
C19  20.7,46.36 0 top
C20  20.7,48.9 0 top
C21  5.59,49.66 0 top
D1  30.23,22.99 90 top
D2  32.26,22.99 90 top
D3  5.71,56.64 0 top
DAC4  25.15,10.03 0 top
FB1  18.8,28.96 180 top
J1  4.83,30.86 270 top
J2  11.3,11.18 0 top
J3  6.48,60.07 0 top
R1  30.23,25.4 270 top
R2  32.26,25.4 270 top
R3  28.83,45.97 90 top
R4  30.99,48.13 270 top
R5  30.99,46.1 90 top
R6  5.71,54.36 0 top
R7  19.94,30.61 0 top
R8  18.54,36.7 180 top
R9  5.71,52.58 0 top
R10  51.94,51.56 90 top
R14  49.28,51.56 90 top
R15  64.14,49.28 90 top
R16  66.55,49.28 90 top
S1  5.46,43.94 90 top
SPI1  40.77,10.92 180 top
U1  31.75,35.69 0 top
U2  31.75,10.16 180 top
U3  58.55,54.1 0 top
U$1  27.05,63.75 0 top
U$2  60.07,11.81 270 top
USART1  49.28,41.15 270 top
USART2  21.97,10.03 180 top
USART3  50.04,20.32 90 top
USART4  27.05,54.61 0 top
Y1  15.49,45.34 90 top
Y2  21.21,40.51 0 top

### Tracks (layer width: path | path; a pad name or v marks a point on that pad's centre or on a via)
3V3  (via drill 0.35)
  Top 0.203: 22.73,43.18 22.73,39.37 22.92,39.19 U1.6 25.73,39.19 v25.78,39.24 | 22.73,43.18 v23.5,43.94 24.26,44.7 | 24.26,44.7 24.26,45.48 C6.1 25.26,47.73 v25.27,47.75 | U1.50 37.75,27.78 39.97,25.57 C12.1 39.97,23.84 39.62,23.49 35.31,23.49 35.18,23.62 35.18,24.49 C8.1 v33.91,24.51 | U1.75 41.18,41.69 42.02,42.53 C9.1 40.64,43.93 40.64,43.94 39.88,43.94 | 39.88,43.94 39.86,43.94 C10.1 38.75,44.81 37.59,45.97 36.72,45.97 C11.1 v36.7,45.21 | 39.88,43.94 v39.5,43.56 | FB1.2 v16.26,28.96 | v32.26,47.75 31.04,47.75 R4.2 R5.2 31.04,46.48 v32,46.48 | C7.1 22.23,43.69 22.73,43.18 | U1.100 25.78,43.57 25.78,44.58 25.15,45.21 24.77,45.21 24.26,44.7 | U1.28 26.8,27.79 v26.8,25.65 | U2.4 30.32,14.82 v30.35,14.86 | C5.1 6.6,21.34 v5.46,22.48 | J3.4 14.1,59.18 v13.21,58.29 | R9.2 v7.11,52.58 | R6.2 v7.11,54.36 | U1.73 41.99,40.69 v42.04,40.64 | U1.11 25.77,36.69 v25.78,36.7 | C4.1 10.88,22.52 v10.86,22.54 | U3.14 62.85,56.15 v62.87,56.13 | U$2.P$4 57.87,18.58 v57.78,18.67
  pour Route15: 0.76,65.66 69.85,65.66 69.85,0.76 0.76,0.76
5V  (via drill 0.35)
  Top 0.203: U2.1 v33.19,8.25 | U2.6 30.32,7.96 29.97,7.62 v29.72,7.62 | J2.3 v8.76,5.59 | J3.3 v11.56,57.91 | C2.1 v14.86,20.95 | C3.1 v5.71,18.41 | U$1.1 v22.73,63.75
  Bottom 0.203: 12.19,20.07 12.19,42.05 11.56,42.68 v11.56,57.91 11.56,62.61 12.7,63.75 v22.73,63.75 | 12.19,20.07 12.19,19.3 9.53,16.64 6.48,16.64 5.71,17.4 v5.71,18.41 4.19,16.89 4.19,7.24 5.97,5.46 8.89,5.46 | v8.76,5.59 8.89,5.46 | 8.89,5.46 10.16,4.19 26.8,4.19 29.59,6.98 | v29.72,7.62 29.72,7.11 29.59,6.98 | v14.86,20.95 13.08,20.95 12.19,20.07 | v33.19,8.25 31.91,6.98 29.59,6.98
  pour Bottom: 1.14,65.66 69.85,65.66 69.85,0.63 0.89,0.63 0.89,65.79 1.14,65.79
5V_IN
  Top 0.203: J3.2 9.02,61.34 | J1.1 5.3,32.16 5.33,32.13 5.97,32.77 5.97,35.69 5.59,36.07 1.4,36.07 1.14,36.32 1.14,61.09 2.29,62.23 8.13,62.23 9.02,61.34 | U$1.2 28.12,64.78 23.65,64.78 23.25,64.39 10.92,64.39 9.02,62.48 9.02,61.34
CS  (via drill 0.35)
  Top 0.203: U1.51 42.32,29.69 v42.42,29.59 | v63.63,41.27 63.88,41.53 63.88,48.37 R15.1
  Bottom 0.203: v42.42,29.59 46.99,29.59 56.9,39.5 62.99,39.5 63.63,40.13 v63.63,41.27
CS_LLS  (via drill 0.35)
  Top 0.203: U$2.P$2 60.07,17.02 60.45,17.4 v60.45,18.92 | U3.6 53.95,52.8 53.34,52.2 53.34,45.72 54.74,44.32 54.74,28.32 v55.37,27.69
  Bottom 0.203: v55.37,27.69 60.45,22.61 v60.45,18.92
D0_LLS
  Top 0.203: U$2.P$7 55.07,15.12 55.07,14.72 55.22,14.57 61.63,14.57 66.29,19.23 66.29,48.37 R16.1
DI_LLS
  Top 0.203: U$2.P$3 58.97,17.82 59.69,18.54 59.69,22.23 56.77,25.15 56.77,54.61 56.63,54.75 U3.3
GND  (via drill 0.35)
  Top 0.203: J1.5 4.86,29.59 v6.22,29.59 | v10.03,6.98 J2.5 J2.7 v11.3,6.86 | U1.20 23.86,32.15 22.48,32.15 21.97,32.66 | U1.19 23.87,32.66 21.97,32.66 | 21.97,32.66 C15.2 19.05,34.05 v19.05,34.16 20.36,34.16 C1.1 | U1.99 26.25,46.43 C6.2 v27.43,46.48 28.75,46.48 R3.2 28.83,49.53 | C12.2 38.14,24.51 37.85,24.51 | 37.85,24.51 C8.2 34.81,25.91 v33.91,25.91 33.66,25.91 33.27,25.53 33.27,22.86 33.02,22.61 32.33,22.61 D2.C 32.26,20.95 31.24,19.94 | U1.74 41.57,41.19 42.67,42.29 42.67,43.05 42.15,43.58 C9.2 42.02,43.58 39.73,45.86 | C10.2 39.73,45.86 | 39.73,45.86 v38.61,46.99 36.72,46.99 C11.2 | C14.C 23.07,23.54 23.11,23.49 v23.05,23.43 | C16.C 13.97,31.88 | 13.97,31.88 v13.97,30.1 | D1.C 30.23,20.95 31.24,19.94 | 31.24,19.94 v31.24,18.8 | C18.2 v11.56,41.78 11.56,42.67 | C17.2 21.07,52.85 21.84,52.07 | 21.84,52.07 v22.86,52.07 26.29,52.07 28.83,49.53 | 21.84,52.07 21.72,52.07 21.23,51.58 C20.2 C19.2 21.23,45.1 19.94,43.82 v19.81,43.82 20.81,43.82 C7.2 | S1.3 9.83,40.94 11.56,42.67 | 11.56,42.67 11.56,44.78 9.88,46.46 | U2.2 U2.7 31.24,10.67 v31.24,12.57 | 28.83,49.53 29.34,50.04 v29.34,51.05 | U1.10 21.74,37.19 20.83,38.1 v20.45,38.1 | U1.49 37.25,25.62 37.85,25.02 37.85,24.51 | J2.11 13.84,8 13.72,7.87 v13.72,6.98 | C3.2 9.4,18.41 10.16,19.18 10.16,20.95 9.78,21.34 C5.2 9.16,22.73 10.69,24.26 12.41,24.26 C4.2 C2.2 v14.86,26.42 | J3.1 6.48,59.31 5.33,58.17 4.57,58.17 | 4.57,58.17 3.3,58.17 v3.17,58.04 | v6.1,51.18 6.1,49.67 C21.2 7.49,49.66 9.88,47.27 9.88,46.46 | D3.C 5.26,57.47 4.57,58.17 | J3.14 J3.13 v36.96,57.91 | v26.04,24.89 26.16,25.02 26.16,25.92 26.25,26 U1.27 | S1.4 7.71,46.99 9.35,46.99 9.88,46.46
  Top 0.203: 13.97,31.88 14.88,32.78 C13.2 17.27,33.4 16.89,33.78 v16.76,33.78 | U$2.P$6 55.67,19.22 v55.75,19.3 52.58,19.3 51.22,17.95 51.22,15.37 | U3.1 v55.62,57.53 v55.63,57.53 | U3.4 v54.23,54.1 | U3.7 54.37,52.05 v54.36,52.07 | U3.13 63.34,55.4 v63.38,55.36 | U3.10 62.37,53.45 v63.25,52.58 | U$2.P$10 51.22,15.37 | U$2.P$13 51.48,15.11 51.22,15.37 | U$2.P$12 66.72,13.45 U$2.P$11 68.33,16.86 v68.33,19.18
  pour Route2: 0.76,65.66 69.85,65.66 69.85,0.89 0.76,0.89
MISO  (via drill 0.35)
  Top 0.203: U1.53 39.63,30.66 40.69,30.66 41.15,31.12 v42.55,31.12 | v64.64,52.19 62.73,54.1 U3.11
  Bottom 0.203: v42.55,31.12 46.74,31.12 65.41,49.78 65.41,51.44 v64.65,52.19 v64.64,52.19
MOSI  (via drill 0.35)
  Top 0.203: U1.54 39.7,31.28 40.3,31.28 40.45,31.43 40.45,31.44 v40.89,31.88 | R14.1 49.28,46.23 46.86,43.82 v46.86,36.7
  Bottom 0.203: v46.86,36.7 45.34,35.18 42.16,35.18 40.89,33.91 v40.89,31.88
N$1
  Top 0.203: R2.1 32.25,25.84 U1.39
N$2
  Top 0.203: R1.1 30.23,26.54 30.48,26.8 31.11,26.8 31.25,26.93 U1.37
N$3
  Top 0.203: D1.A R1.2
N$4
  Top 0.203: D2.A R2.2
N$5
  Top 0.203: U1.94 28.75,45.46 R3.1
N$6
  Top 0.203: U1.93 29.25,45 29.59,45.34 29.59,47.88 30.28,48.57 R4.1
N$7
  Top 0.203: U1.92 29.75,44.99 30.43,45.67 R5.1
N$8
  Top 0.203: D3.A 7.24,56.64 7.49,56.39 7.49,55.88 7.11,55.5 5.97,55.5 5.28,54.81 R6.1
N$9  (via drill 0.35)
  Top 0.203: U1.33 29.25,26.69 v29.1,26.54 | v48.64,24.13 48.77,24.13 USART3.2
  Bottom 0.203: v29.1,26.54 v29.11,26.54 46.23,26.54 v48.64,24.13
N$10
  Top 0.203: C1.2 22.48,34.25 22.48,33.4 22.69,33.19 U1.18
N$11  (via drill 0.35)
  Top 0.203: U1.34 29.75,26.77 29.84,26.67 29.84,26.38 29.67,26.21 29.67,25.84 v29.23,25.4 | v48.13,20.32 USART3.1
  Bottom 0.203: v29.23,25.4 29.23,21.45 30.35,20.32 v48.13,20.32
N$12
  Top 0.203: C18.1 11.56,38.99 | 11.56,38.99 11.56,37.97 12.19,37.34 15.24,37.34 15.88,36.7 R8.2 | 11.56,38.99 12.06,38.48 13.39,38.48 Y1.1
N$13
  Top 0.203: R14.2 49.28,54.36 50.32,55.4 U3.2
N$14  (via drill 0.35)
  Top 0.203: USART4.2 30.86,53.34 v30.86,52.7 | v35.43,45.59 36.07,44.95 36.75,44.27 U1.78
  Bottom 0.203: v30.86,52.7 30.86,52.07 35.31,47.62 35.31,45.72 v35.43,45.59
N$15  (via drill 0.35)
  Top 0.203: U1.29 27.25,26.09 27.43,25.92 27.43,25.14 26.04,23.75 v26.04,21.84 | DAC4.1 25.02,10.16 25.02,12.57 25.65,13.21 v26.04,13.21
  Bottom 0.203: v26.04,21.84 v26.04,13.21
N$16  (via drill 0.35)
  Top 0.203: U1.79 36.15,43.63 36.15,44.24 35.56,44.83 v34.67,44.83 | v27.56,52.32 27.05,52.83 USART4.1
  Bottom 0.203: v34.67,44.83 33.4,46.1 33.4,48.64 29.72,52.32 v27.56,52.32
N$17  (via drill 0.35)
  Top 0.203: U1.30 27.75,26.1 27.79,26.06 27.79,19.84 v27.81,19.81 | v36.39,11.24 37.91,11.24 SPI1.2
  Bottom 0.203: v27.81,19.81 v36.39,11.24 36.45,11.18
N$18  (via drill 0.35)
  Top 0.203: U1.31 28.35,27.74 28.35,27.13 28.45,27.03 28.45,20.07 28.57,19.94 v28.72,19.94 | v40.26,13.08 40.77,12.57 SPI1.1
  Bottom 0.203: v28.72,19.94 35.58,13.08 v40.26,13.08
N$19  (via drill 0.35)
  Top 0.203: U1.69 39.65,38.73 v41.53,38.73 | v49.28,43.31 USART1.1
  Bottom 0.203: v41.53,38.73 46.1,43.31 v49.28,43.31
N$20  (via drill 0.35)
  Top 0.203: U1.68 41.06,38.19 v41.66,37.59 | v47.75,39.88 48.01,39.88 USART1.2
  Bottom 0.203: v41.66,37.59 43.94,39.88 v47.75,39.88
N$22  (via drill 0.35)
  Top 0.203: U1.25 22.63,29.69 v22.48,29.84 | v19.43,12.57 USART2.2
  Bottom 0.203: v22.48,29.84 22.48,23.75 22.42,23.69 22.42,21.15 19.43,18.16 v19.43,12.57
N$23  (via drill 0.35)
  Top 0.203: U1.26 25.27,27.36 v25.27,26.03 | v21.97,12.45 USART2.1
  Bottom 0.203: v25.27,26.03 25.27,19.69 21.97,16.38 v21.97,12.45
N$24
  Top 0.203: R10.2 53.18,53.45 U3.5
N$25
  Top 0.203: U3.9 61.67,52.61 62.25,52.61 64.14,50.72 R15.2
N$26
  Top 0.203: U3.12 62.98,54.75 66.55,51.18 R16.2
NRST
  Top 0.203: U1.14 21.71,35.19 21.21,35.69 16.26,35.69 14.99,36.96 9.53,36.96 | S1.1 3.43,41.16 3.43,37.97 | 9.53,36.96 4.45,36.96 3.43,37.97 | 3.43,37.97 2.54,38.86 1.91,38.86 1.52,39.24 1.52,46.82 1.65,46.94 S1.2 3.43,47.16 3.43,48.77 | 3.43,48.77 4.32,49.66 C21.1 | 3.43,48.77 3.43,51.94 4.06,52.58 R9.1 5.33,52.63 5.33,53.34 5.59,53.59 10.16,53.59 J3.5 | J2.12 13.84,11.3 14.48,10.67 14.48,4.93 13.34,3.79 2.44,3.79 1.91,4.32 1.91,24.38 2.79,25.27 4.83,25.27 7.62,28.07 7.62,35.05 9.53,36.96
PC14-OSC32-IN
  Top 0.203: U1.8 22.77,38.19 21.84,39.12 21.84,40.45 Y2.2 21.91,42.1 21.34,42.67 19.05,42.67 18.8,42.93 18.8,45.85 19.3,46.36 C19.1
PC15-OSC32-OUT
  Top 0.203: U1.9 22.13,37.69 20.51,39.31 Y2.1 20.51,40.96 20.45,41.02 20.45,41.53 19.81,42.16 18.67,42.16 18.29,42.55 18.29,48.13 19.05,48.9 C20.1
PH0-OSC-IN
  Top 0.203: U1.12 21.85,36.19 20.83,37.21 19.68,37.21 16.89,40.01 16.89,45.85 | C17.1 18.92,51.69 18.16,50.93 17.27,50.93 16.89,50.55 16.89,45.85 | 16.89,45.85 16.26,46.48 15.88,46.48 15.49,46.86 Y1.2
PH1-OSC-OUT
  Top 0.203: U1.13 21.72,35.69 20.7,36.7 R8.1
SCK  (via drill 0.35)
  Top 0.203: U1.52 39.7,30.28 41.33,30.28 v41.53,30.48 | v51.94,49.4 R10.1
  Bottom 0.203: v41.53,30.48 41.53,31.62 43.81,33.91 47.62,33.91 51.94,38.23 v51.94,49.4
SCK_LLS  (via drill 0.35)
  Top 0.203: U$2.P$5 56.77,21.08 54.74,23.11 v54.74,25.53 | U3.8 61.47,37.6 58.42,34.54 v58.29,34.54
  Bottom 0.203: v58.29,34.54 55.5,31.75 52.32,31.75 50.93,30.35 50.93,27.94 53.34,25.53 v54.74,25.53
SWCLK  (via drill 0.35)
  Top 0.203: J2.9 12.57,6.48 11.68,5.59 10.16,5.59 9.4,6.35 9.4,10.67 9.02,11.05 8.76,11.05 8.13,11.68 8.13,14.86 8.26,14.99 9.91,14.99 10.03,14.86 J2.6 10.03,11.28 10.16,11.15 11.4,11.15 11.94,11.68 11.94,19.18 v11.3,19.81 | v10.41,52.7 12.45,54.74 18.29,54.74 21.08,57.53 v30.48,57.53 | v37.72,44.83 37.75,44.8 U1.76
  Bottom 0.203: v11.3,19.81 10.79,20.32 10.79,21.34 9.78,22.35 9.78,52.07 v10.41,52.7 | v30.48,57.53 35.69,57.53 40.64,52.58 45.34,52.58 47.5,50.42 47.5,47.88 46.99,47.37 40.64,47.37 40.13,47.88 38.1,47.88 37.72,47.5 v37.72,44.83
SWDIO
  Top 0.203: U1.72 41.35,40.19 42.8,38.73 42.93,38.61 43.18,38.35 43.18,20.57 40.39,17.78 15.11,17.78 14.73,17.4 14.48,17.14 13.21,15.88 13.21,11.68 12.32,10.79 9.78,10.79 8.76,11.81 J2.4
SWO  (via drill 0.35)
  Top 0.203: 14.86,27.4 v14.86,27.43 7.75,27.43 3.94,23.62 3.94,18.03 4.7,17.27 10.54,17.27 11.3,16.5 J2.8 | v31.24,44.58 v31.25,44.57 U1.89
  Bottom 0.203: v14.86,27.43 14.86,29.46 15.88,30.48 15.88,34.93 16.26,35.31 19.05,35.31 19.68,35.94 19.68,38.86 18.41,40.13 18.41,46.36 19.94,47.88 23.75,47.88 25.02,49.15 28.32,49.15 29.97,47.5 29.97,45.09 30.48,44.58 v31.24,44.58
USART_RX  (via drill 0.35)
  Top 0.203: U1.87 32.25,45.71 32.89,46.35 v32.89,50.92 v32.89,50.93 31.88,51.94 J3.11 | v45.72,48.64 45.72,6.98 44.45,5.71 16.26,5.71 15.11,6.86 J2.13
  Bottom 0.203: v32.89,50.93 43.43,50.93 v45.72,48.64
USART_TX
  Top 0.203: U1.86 32.75,44.82 34.42,46.48 34.42,57.02 | J3.12 34.42,57.02 | 34.42,57.02 44.58,46.86 44.58,17.53 42.93,15.88 17.78,15.88 J2.14
VDDA
  Top 0.203: FB1.1 19.94,28.96 | 19.94,28.96 20.57,28.96 21.59,29.97 21.59,30.73 22.04,31.19 U1.22 | FB1.1 17.27,31.28 C13.1 | FB1.1 19.6,29.76 20.37,30.53 R7.2 | C14.A 19.94,25.83 19.94,28.96
VREF_PLUS
  Top 0.203: U1.21 23.82,31.61 C15.1 20.07,31.61 | 20.07,31.61 19.96,31.61 16.81,34.75 C16.A | R7.1 19.51,31.05 20.07,31.61

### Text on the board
tPlace: Smart Home Assistant PCB V1 | Logan Geivet, Peter Lototsky, Jackson Newman, / Nicholas Pellegrin, and Alexander Robles

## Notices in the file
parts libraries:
SparkFun-Connectors: Licensing: Creative Commons ShareAlike 4.0 International - https://creativecommons.org/licenses/by-sa/4.0
